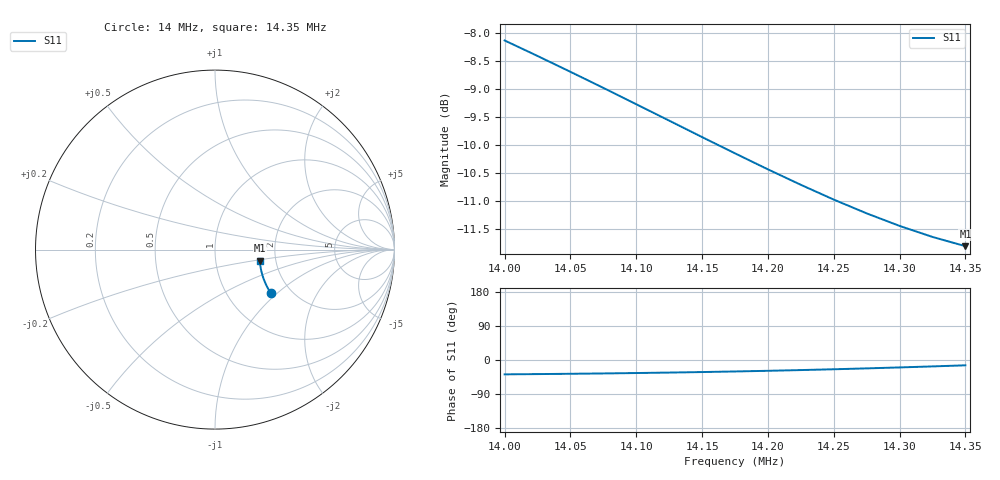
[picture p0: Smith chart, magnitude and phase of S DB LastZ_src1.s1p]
! EZNEC Pro/4 beta ver. A6.0
! 5/17/2015 1:02:05 PM
! Back yard dipole
! Source 1
# MHZ S DB R 50
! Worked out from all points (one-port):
!   15 points, 14 MHz to 14.35 MHz, reference 50 ohm
!   lowest |S11| = -11.8 dB at 14.35 MHz (marker M1), VSWR 1.69, Z = 82.3 - j11 ohm
!   |S11| at or under -10 dB: 14.163 MHz to end of sweep
14  -8.12 -37.9
14.025  -8.40 -37.2
14.05  -8.69 -36.4
14.075  -8.97 -35.5
14.1  -9.26 -34.4
14.125  -9.56 -33.2
14.15  -9.85 -31.8
14.175  -10.14 -30.3
14.2  -10.43 -28.5
14.225  -10.70 -26.6
14.25  -10.97 -24.5
14.275  -11.21 -22.1
14.3  -11.44 -19.6
14.325  -11.63 -16.9
14.35  -11.80 -14.1
